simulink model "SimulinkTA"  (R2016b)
settings: Solver=VariableStepAuto  StartTime=0.0  StopTime=10000  RelTol=1e-3
libraries: simulink x15, sldrtlib x1
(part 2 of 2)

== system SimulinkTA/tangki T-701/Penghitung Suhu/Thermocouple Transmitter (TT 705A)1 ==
  note: mA
  In1 : Inport  RequirementInfo={} %GIDa_a3a1ad45_919b_4aba_9b26_8d553a2688f7
  Bias : Bias  RequirementInfo={} %GIDa_1c3de125_1f5d_410d_80ff_796fe57e2ba6  Bias=4
  Thermocouple Transmitter Transfer Function : TransferFcn  RequirementInfo={} %GIDa_91057ead_186f_4539_8c2c_8d461ed5b72a  Numerator=[0.16]  Denominator=[2 1]
  Out1 : Outport  RequirementInfo={} %GIDa_260862c9_6f60_4f64_adb1_f88b03570b65
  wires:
  Bias/1 -> Out1/1
  In1/1 -> Thermocouple Transmitter Transfer Function/1
  Thermocouple Transmitter Transfer Function/1 -> Bias/1
